FUNCTION "CAMB_PACCO" : VOID
TITLE =
AUTHOR : D_T
VERSION : 0.1

BEGIN
NETWORK
TITLE =pulsante luminoso Cambio pacco prenotato
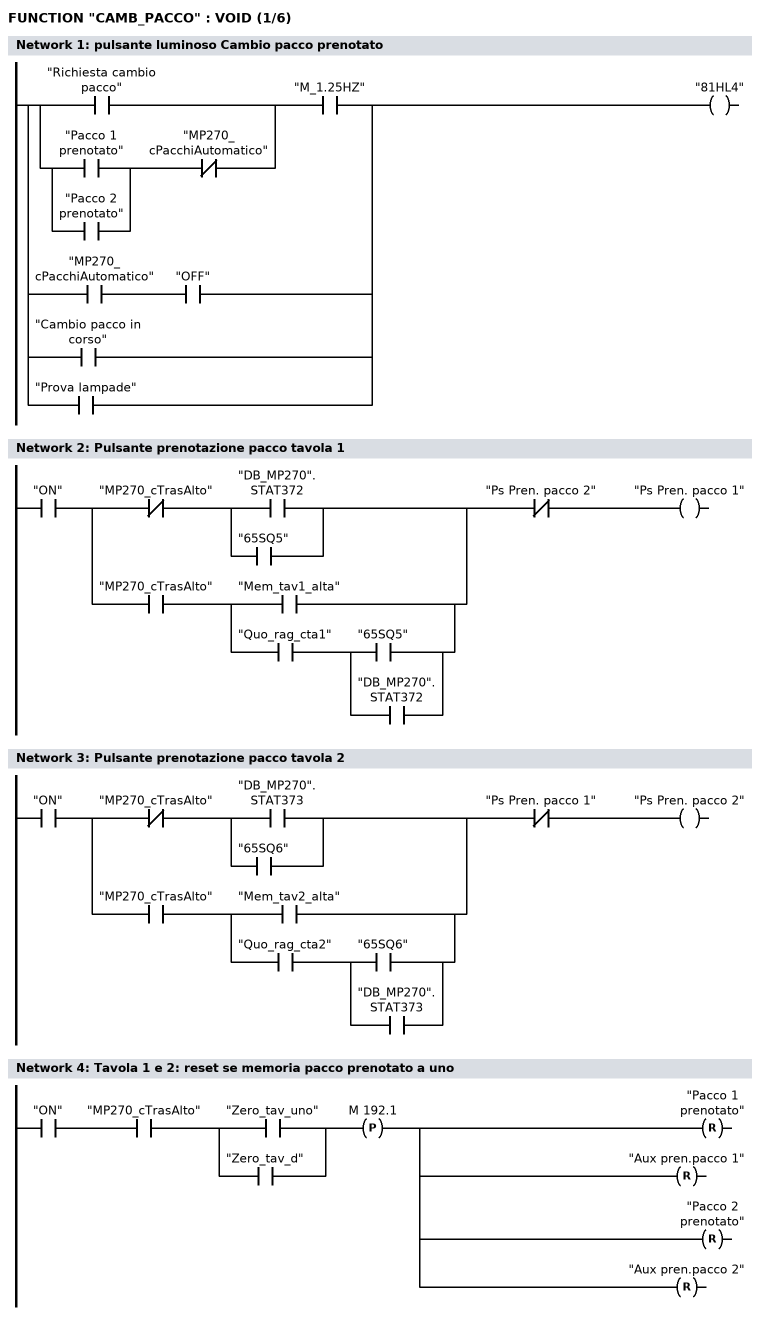
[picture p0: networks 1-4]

      U(    ;
      O     "Richiesta cambio pacco";
      O     ;
      U(    ;
      O     "Pacco 1 prenotato";
      O     "Pacco 2 prenotato";
      )     ;
      UN    "MP270_cPacchiAutomatico";
      )     ;
      U     "M_1.25HZ";
      O     ;
      U     "MP270_cPacchiAutomatico";
      U     "OFF";
      O     "Cambio pacco in corso";
      O     "Prova lampade";
      =     "81HL4";
NETWORK
TITLE =Pulsante prenotazione pacco tavola 1

      U     "ON";
      U(    ;
      UN    "MP270_cTrasAlto";
      U(    ;
      O     "DB_MP270".STAT372;
      O     "65SQ5";
      )     ;
      O     ;
      U     "MP270_cTrasAlto";
      U(    ;
      O     "Mem_tav1_alta";
      O     ;
      U     "Quo_rag_cta1";
      U(    ;
      O     "65SQ5";
      O     "DB_MP270".STAT372;
      )     ;
      )     ;
      )     ;
      UN    "Ps Pren. pacco 2";
      =     "Ps Pren. pacco 1";
NETWORK
TITLE =Pulsante prenotazione pacco tavola 2

      U     "ON";
      U(    ;
      UN    "MP270_cTrasAlto";
      U(    ;
      O     "DB_MP270".STAT373;
      O     "65SQ6";
      )     ;
      O     ;
      U     "MP270_cTrasAlto";
      U(    ;
      O     "Mem_tav2_alta";
      O     ;
      U     "Quo_rag_cta2";
      U(    ;
      O     "65SQ6";
      O     "DB_MP270".STAT373;
      )     ;
      )     ;
      )     ;
      UN    "Ps Pren. pacco 1";
      =     "Ps Pren. pacco 2";
NETWORK
TITLE =Tavola 1 e 2: reset se memoria pacco prenotato a uno

      U     "ON";
      U     "MP270_cTrasAlto";
      U(    ;
      O     "Zero_tav_uno";
      O     "Zero_tav_d";
      )     ;
      FP    M    192.1;
      R     "Pacco 1 prenotato";
      R     "Aux pren.pacco 1";
      R     "Pacco 2 prenotato";
      R     "Aux pren.pacco 2";
NETWORK
TITLE =Tavola 1 : Pacco prenotato
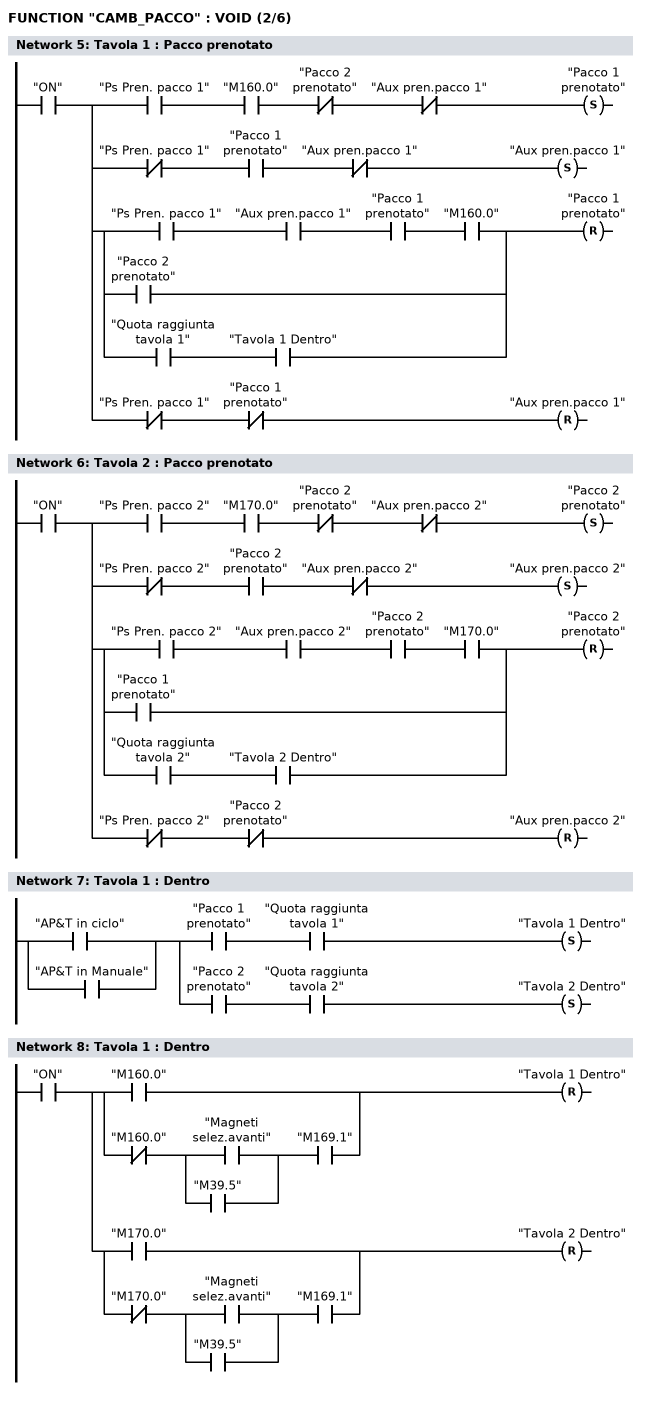
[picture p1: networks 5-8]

      U     "ON";
      =     L      0.0;
      U     L      0.0;
      U     "Ps Pren. pacco 1";
      U     "M160.0";
      UN    "Pacco 2 prenotato";
      UN    "Aux pren.pacco 1";
      S     "Pacco 1 prenotato";
      U     L      0.0;
      UN    "Ps Pren. pacco 1";
      U     "Pacco 1 prenotato";
      UN    "Aux pren.pacco 1";
      S     "Aux pren.pacco 1";
      U     L      0.0;
      U(    ;
      U     "Ps Pren. pacco 1";
      U     "Aux pren.pacco 1";
      U     "Pacco 1 prenotato";
      U     "M160.0";
      O     "Pacco 2 prenotato";
      O     ;
      U     "Quota raggiunta tavola 1";
      U     "Tavola 1 Dentro";
      )     ;
      R     "Pacco 1 prenotato";
      U     L      0.0;
      UN    "Ps Pren. pacco 1";
      UN    "Pacco 1 prenotato";
      R     "Aux pren.pacco 1";
NETWORK
TITLE =Tavola 2 : Pacco prenotato

      U     "ON";
      =     L      0.0;
      U     L      0.0;
      U     "Ps Pren. pacco 2";
      U     "M170.0";
      UN    "Pacco 2 prenotato";
      UN    "Aux pren.pacco 2";
      S     "Pacco 2 prenotato";
      U     L      0.0;
      UN    "Ps Pren. pacco 2";
      U     "Pacco 2 prenotato";
      UN    "Aux pren.pacco 2";
      S     "Aux pren.pacco 2";
      U     L      0.0;
      U(    ;
      U     "Ps Pren. pacco 2";
      U     "Aux pren.pacco 2";
      U     "Pacco 2 prenotato";
      U     "M170.0";
      O     "Pacco 1 prenotato";
      O     ;
      U     "Quota raggiunta tavola 2";
      U     "Tavola 2 Dentro";
      )     ;
      R     "Pacco 2 prenotato";
      U     L      0.0;
      UN    "Ps Pren. pacco 2";
      UN    "Pacco 2 prenotato";
      R     "Aux pren.pacco 2";
NETWORK
TITLE =Tavola 1 : Dentro

      O     "AP&T  in ciclo";
      O     "AP&T in Manuale";
      =     L      0.0;
      U     L      0.0;
      U     "Pacco 1 prenotato";
      U     "Quota raggiunta tavola 1";
      S     "Tavola 1 Dentro";
      U     L      0.0;
      U     "Pacco 2 prenotato";
      U     "Quota raggiunta tavola 2";
      S     "Tavola 2 Dentro";
NETWORK
TITLE =Tavola 1 : Dentro

      U     "ON";
      =     L      0.0;
      U     L      0.0;
      U(    ;
      O     "M160.0";
      O     ;
      UN    "M160.0";
      U(    ;
      O     "Magneti selez.avanti";
      O     "M39.5";
      )     ;
      U     "M169.1";
      )     ;
      R     "Tavola 1 Dentro";
      U     L      0.0;
      U(    ;
      O     "M170.0";
      O     ;
      UN    "M170.0";
      U(    ;
      O     "Magneti selez.avanti";
      O     "M39.5";
      )     ;
      U     "M169.1";
      )     ;
      R     "Tavola 2 Dentro";
NETWORK
TITLE =Tavola 1 : Prenotazione visualizzata su MP270
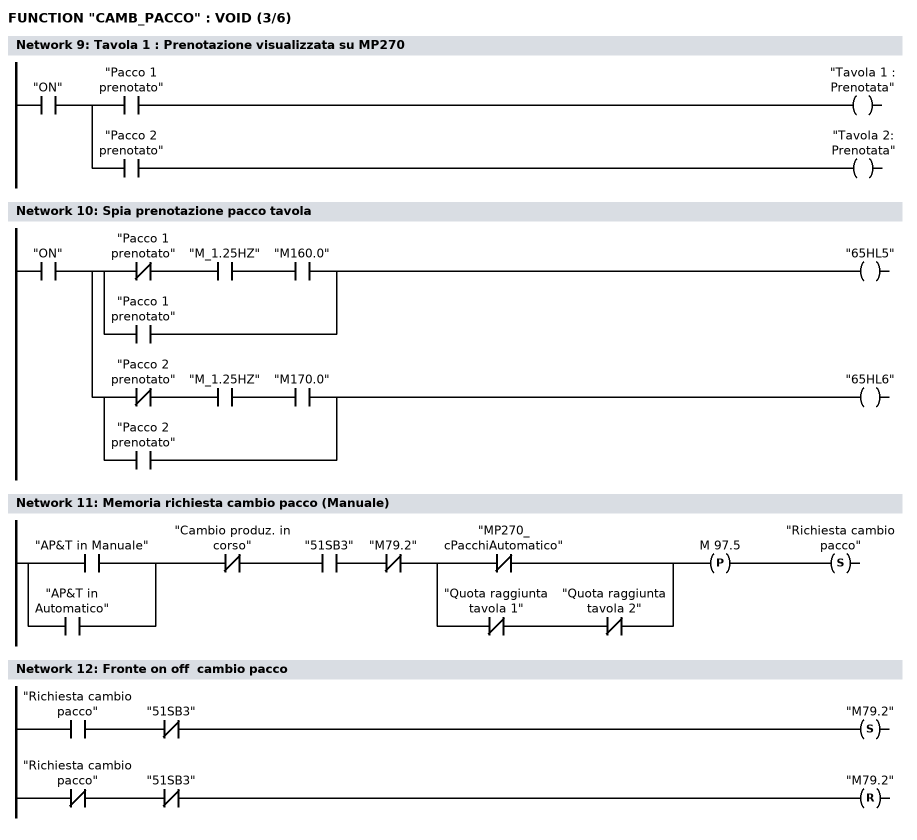
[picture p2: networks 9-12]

      U     "ON";
      =     L      0.0;
      U     L      0.0;
      U     "Pacco 1 prenotato";
      =     "Tavola 1 : Prenotata";
      U     L      0.0;
      U     "Pacco 2 prenotato";
      =     "Tavola 2: Prenotata";
NETWORK
TITLE =Spia prenotazione pacco tavola

      U     "ON";
      =     L      0.0;
      U     L      0.0;
      U(    ;
      UN    "Pacco 1 prenotato";
      U     "M_1.25HZ";
      U     "M160.0";
      O     "Pacco 1 prenotato";
      )     ;
      =     "65HL5";
      U     L      0.0;
      U(    ;
      UN    "Pacco 2 prenotato";
      U     "M_1.25HZ";
      U     "M170.0";
      O     "Pacco 2 prenotato";
      )     ;
      =     "65HL6";
NETWORK
TITLE =Memoria richiesta cambio pacco (Manuale)

      U(    ;
      O     "AP&T in Manuale";
      O     "AP&T in Automatico";
      )     ;
      UN    "Cambio produz. in corso";
      U     "51SB3";
      UN    "M79.2";
      U(    ;
      ON    "MP270_cPacchiAutomatico";
      O     ;
      UN    "Quota raggiunta tavola 1";
      UN    "Quota raggiunta tavola 2";
      )     ;
      FP    M     97.5;
      S     "Richiesta cambio pacco";
NETWORK
TITLE =Fronte on off  cambio pacco

      U     "Richiesta cambio pacco";
      UN    "51SB3";
      S     "M79.2";
      UN    "Richiesta cambio pacco";
      UN    "51SB3";
      R     "M79.2";
      NOP   0;
NETWORK
TITLE =Memoria cambio pacco
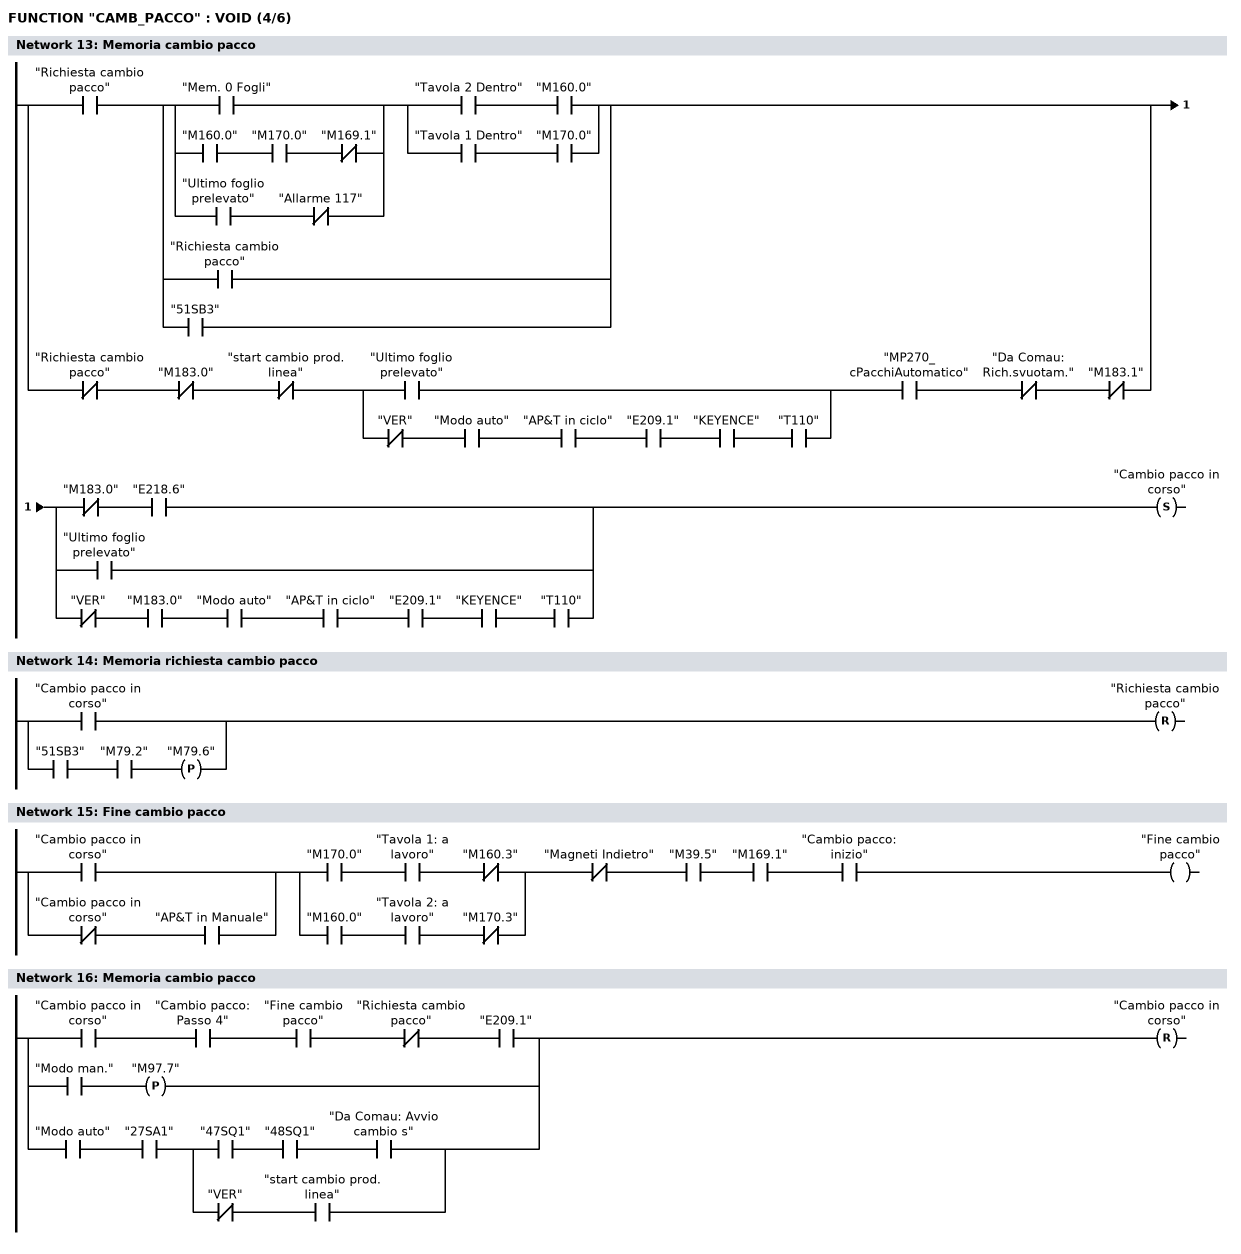
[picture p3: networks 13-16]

      U(    ;
      U     "Richiesta cambio pacco";
      U(    ;
      U(    ;
      O     "Mem. 0 Fogli";
      O     ;
      U     "M160.0";
      U     "M170.0";
      UN    "M169.1";
      O     ;
      U     "Ultimo foglio prelevato";
      UN    "Allarme 117";
      )     ;
      U(    ;
      U     "Tavola 2 Dentro";
      U     "M160.0";
      O     ;
      U     "Tavola 1 Dentro";
      U     "M170.0";
      )     ;
      O     "Richiesta cambio pacco";
      O     "51SB3";
      )     ;
      O     ;
      UN    "Richiesta cambio pacco";
      UN    "M183.0";
      UN    "start cambio prod. linea";
      U(    ;
      O     "Ultimo foglio prelevato";
      O     ;
      UN    "VER";
      U     "Modo auto";
      U     "AP&T  in ciclo";
      U     "E209.1";
      U     "KEYENCE";
      U     "T110";
      )     ;
      U     "MP270_cPacchiAutomatico";
      UN    "Da Comau: Rich.svuotam.";
      UN    "M183.1";
      )     ;
      U(    ;
      UN    "M183.0";
      U     "E218.6";
      O     "Ultimo foglio prelevato";
      O     ;
      UN    "VER";
      U     "M183.0";
      U     "Modo auto";
      U     "AP&T  in ciclo";
      U     "E209.1";
      U     "KEYENCE";
      U     "T110";
      )     ;
      S     "Cambio pacco in corso";
NETWORK
TITLE =Memoria richiesta cambio pacco

      O     "Cambio pacco in corso";
      O(    ;
      U     "51SB3";
      U     "M79.2";
      FP    "M79.6";
      )     ;
      R     "Richiesta cambio pacco";
NETWORK
TITLE =Fine cambio pacco

      U(    ;
      O     "Cambio pacco in corso";
      O     ;
      UN    "Cambio pacco in corso";
      U     "AP&T in Manuale";
      )     ;
      U(    ;
      U     "M170.0";
      U     "Tavola 1: a  lavoro";
      UN    "M160.3";
      O     ;
      U     "M160.0";
      U     "Tavola 2: a  lavoro";
      UN    "M170.3";
      )     ;
      UN    "Magneti Indietro";
      U     "M39.5";
      U     "M169.1";
      U     "Cambio pacco: inizio";
      =     "Fine cambio pacco";
NETWORK
TITLE =Memoria cambio pacco

      U     "Cambio pacco in corso";
      U     "Cambio pacco: Passo 4";
      U     "Fine cambio pacco";
      UN    "Richiesta cambio pacco";
      U     "E209.1";
      O(    ;
      U     "Modo man.";
      FP    "M97.7";
      )     ;
      O     ;
      U     "Modo auto";
      U     "27SA1";
      U(    ;
      U     "47SQ1";
      U     "48SQ1";
      U     "Da Comau: Avvio cambio s";
      O     ;
      UN    "VER";
      U     "start cambio prod. linea";
      )     ;
      R     "Cambio pacco in corso";
NETWORK
TITLE =Cambio pacco: inizio lavoro
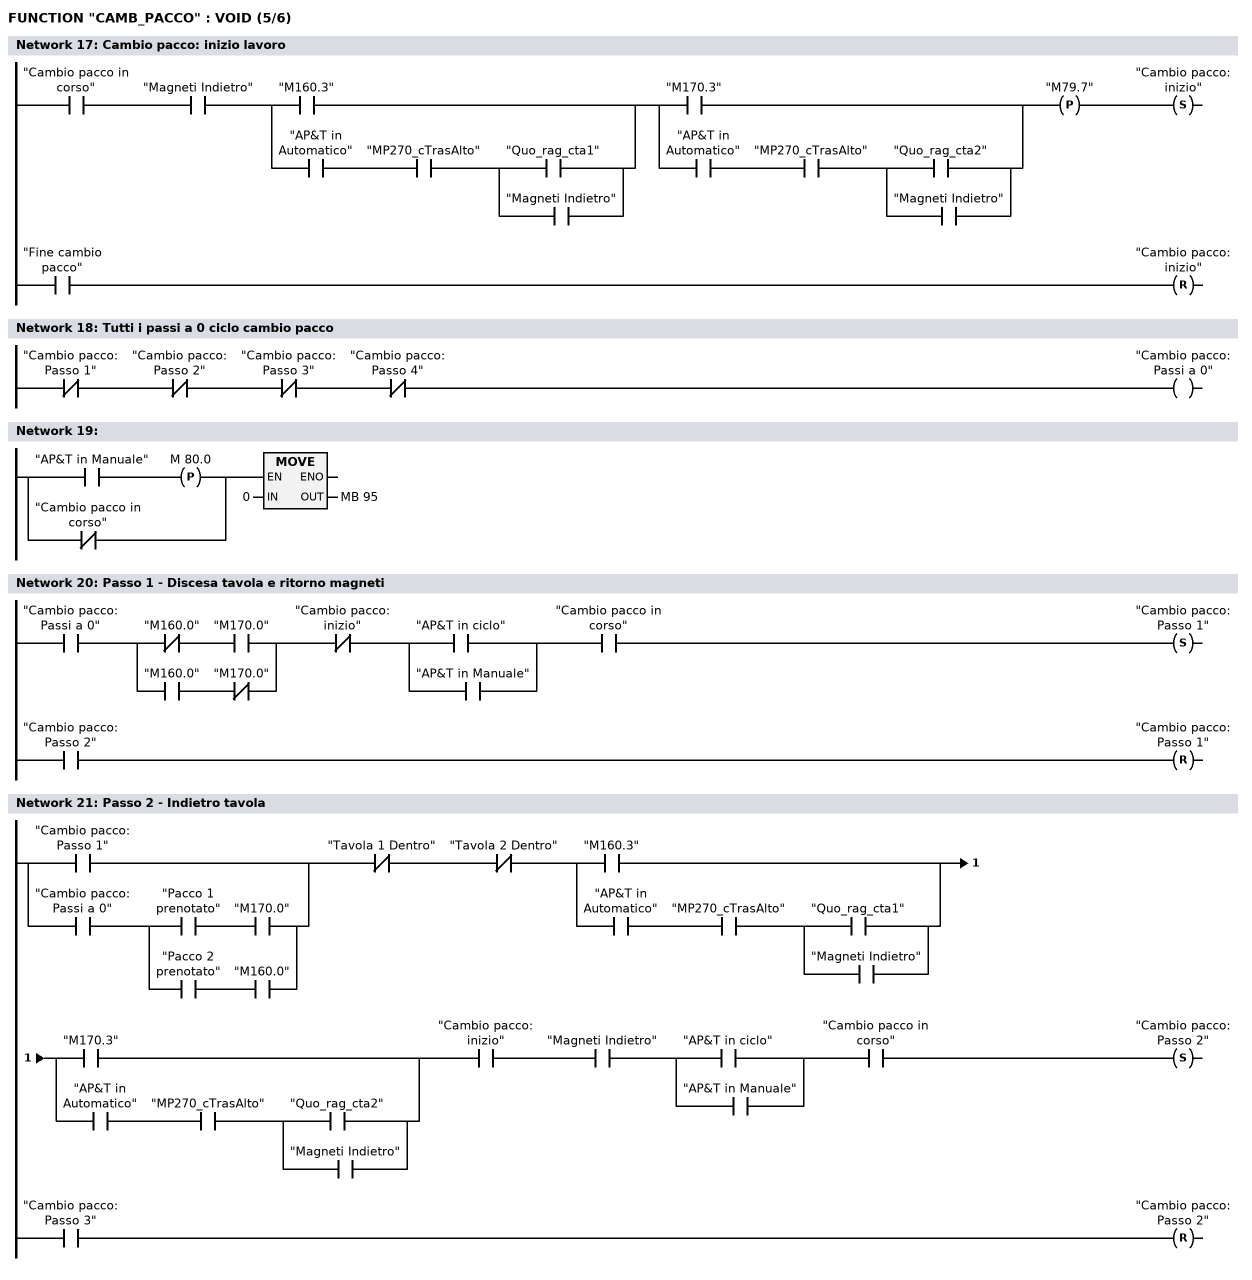
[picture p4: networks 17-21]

      U     "Cambio pacco in corso";
      U     "Magneti Indietro";
      U(    ;
      O     "M160.3";
      O     ;
      U     "AP&T in Automatico";
      U     "MP270_cTrasAlto";
      U(    ;
      O     "Quo_rag_cta1";
      O     "Magneti Indietro";
      )     ;
      )     ;
      U(    ;
      O     "M170.3";
      O     ;
      U     "AP&T in Automatico";
      U     "MP270_cTrasAlto";
      U(    ;
      O     "Quo_rag_cta2";
      O     "Magneti Indietro";
      )     ;
      )     ;
      FP    "M79.7";
      S     "Cambio pacco: inizio";
      U     "Fine cambio pacco";
      R     "Cambio pacco: inizio";
      NOP   0;
NETWORK
TITLE =Tutti i passi a 0 ciclo cambio pacco

      UN    "Cambio pacco: Passo 1";
      UN    "Cambio pacco: Passo 2";
      UN    "Cambio pacco: Passo 3";
      UN    "Cambio pacco: Passo 4";
      =     "Cambio pacco: Passi a 0";
NETWORK
TITLE =

      U(    ;
      U     "AP&T in Manuale";
      FP    M     80.0;
      ON    "Cambio pacco in corso";
      )     ;
      SPBNB _001;
      L     0;
      T     MB    95;
_001: NOP   0;
NETWORK
TITLE =Passo 1 - Discesa tavola e ritorno magneti

      U     "Cambio pacco: Passi a 0";
      U(    ;
      UN    "M160.0";
      U     "M170.0";
      O     ;
      U     "M160.0";
      UN    "M170.0";
      )     ;
      UN    "Cambio pacco: inizio";
      U(    ;
      O     "AP&T  in ciclo";
      O     "AP&T in Manuale";
      )     ;
      U     "Cambio pacco in corso";
      S     "Cambio pacco: Passo 1";
      U     "Cambio pacco: Passo 2";
      R     "Cambio pacco: Passo 1";
      NOP   0;
NETWORK
TITLE =Passo 2 - Indietro tavola

      U(    ;
      O     "Cambio pacco: Passo 1";
      O     ;
      U     "Cambio pacco: Passi a 0";
      U(    ;
      U     "Pacco 1 prenotato";
      U     "M170.0";
      O     ;
      U     "Pacco 2 prenotato";
      U     "M160.0";
      )     ;
      )     ;
      UN    "Tavola 1 Dentro";
      UN    "Tavola 2 Dentro";
      U(    ;
      O     "M160.3";
      O     ;
      U     "AP&T in Automatico";
      U     "MP270_cTrasAlto";
      U(    ;
      O     "Quo_rag_cta1";
      O     "Magneti Indietro";
      )     ;
      )     ;
      U(    ;
      O     "M170.3";
      O     ;
      U     "AP&T in Automatico";
      U     "MP270_cTrasAlto";
      U(    ;
      O     "Quo_rag_cta2";
      O     "Magneti Indietro";
      )     ;
      )     ;
      U     "Cambio pacco: inizio";
      U     "Magneti Indietro";
      U(    ;
      O     "AP&T  in ciclo";
      O     "AP&T in Manuale";
      )     ;
      U     "Cambio pacco in corso";
      S     "Cambio pacco: Passo 2";
      U     "Cambio pacco: Passo 3";
      R     "Cambio pacco: Passo 2";
      NOP   0;
NETWORK
TITLE =Passo 3 - Salita tavola
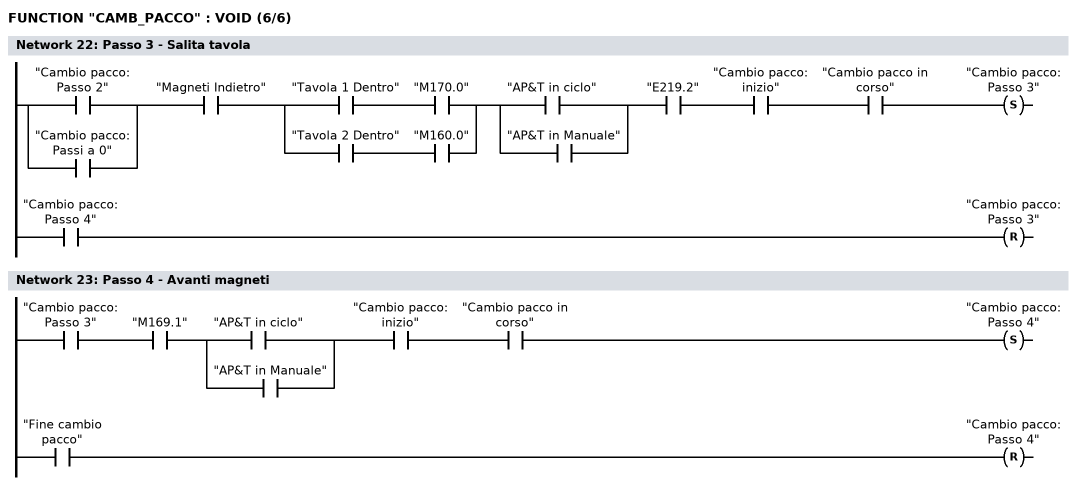
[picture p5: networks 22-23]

      U(    ;
      O     "Cambio pacco: Passo 2";
      O     "Cambio pacco: Passi a 0";
      )     ;
      U     "Magneti Indietro";
      U(    ;
      U     "Tavola 1 Dentro";
      U     "M170.0";
      O     ;
      U     "Tavola 2 Dentro";
      U     "M160.0";
      )     ;
      U(    ;
      O     "AP&T  in ciclo";
      O     "AP&T in Manuale";
      )     ;
      U     "E219.2";
      U     "Cambio pacco: inizio";
      U     "Cambio pacco in corso";
      S     "Cambio pacco: Passo 3";
      U     "Cambio pacco: Passo 4";
      R     "Cambio pacco: Passo 3";
      NOP   0;
NETWORK
TITLE =Passo 4 - Avanti magneti

      U     "Cambio pacco: Passo 3";
      U     "M169.1";
      U(    ;
      O     "AP&T  in ciclo";
      O     "AP&T in Manuale";
      )     ;
      U     "Cambio pacco: inizio";
      U     "Cambio pacco in corso";
      S     "Cambio pacco: Passo 4";
      U     "Fine cambio pacco";
      R     "Cambio pacco: Passo 4";
      NOP   0;
END_FUNCTION

